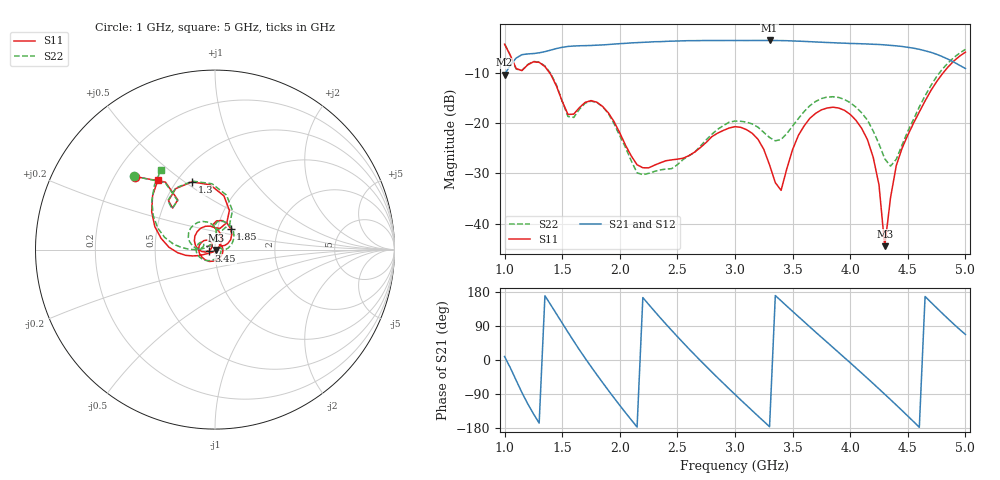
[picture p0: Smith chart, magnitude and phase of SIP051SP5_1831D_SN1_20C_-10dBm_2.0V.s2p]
# GHz  S  dB  R  50
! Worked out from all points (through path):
!   81 points, 1 GHz to 5 GHz, reference 50 ohm
!   highest |S21| = -3.65 dB at 3.3 GHz (marker M1); lowest = -10.4 dB at 1 GHz (marker M2)
!   lowest |S11| = -44.4 dB at 4.3 GHz (marker M3), VSWR 1.01, Z = 50.5 - j0.265 ohm
!   |S11| at or under -10 dB: 1.388 GHz to 4.81 GHz (3.421 GHz wide, 110 % of centre)
!   |S22| runs from -30.3 to -4.3 dB; largest |S21 - S12| = 0.0028
!   S11 on the Smith chart (normalised r, x): 1 GHz: 0.28, +0.36; 1.3 GHz: 0.59, +0.53; 1.85 GHz: 1.15, +0.28; 3.45 GHz: 0.93, -0.01; 5 GHz: 0.40, +0.41
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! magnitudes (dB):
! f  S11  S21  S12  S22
! 1 GHz  -4.4  -10.4  -10.4  -4.3
! 1.1 GHz  -9.2  -7.1  -7.1  -9.3
! 1.3 GHz  -8.0  -6.1  -6.1  -7.9
! 1.55 GHz  -18.3  -4.8  -4.8  -18.7
! 1.7 GHz  -15.9  -4.7  -4.7  -16.1
! 1.85 GHz  -16.7  -4.5  -4.5  -16.7
! 2.15 GHz  -28.3  -4.1  -4.1  -29.9
! 2.35 GHz  -27.9  -3.9  -3.9  -29.3
! 3 GHz  -20.7  -3.7  -3.6  -19.6
! 3.2 GHz  -23.2  -3.7  -3.7  -20.8
! 3.3 GHz  -28.3  -3.6  -3.7  -22.9
! 3.4 GHz  -33.4  -3.7  -3.7  -23.3
! 3.45 GHz  -29.1  -3.7  -3.7  -22.1
! 3.7 GHz  -18.1  -3.9  -3.9  -15.7
! 3.9 GHz  -17.0  -4.2  -4.2  -14.9
! 4.1 GHz  -21.1  -4.3  -4.3  -18.0
! 4.25 GHz  -32.3  -4.4  -4.5  -24.2
! 4.3 GHz  -44.4  -4.5  -4.5  -27.1
! 4.35 GHz  -34.8  -4.6  -4.6  -28.6
! 4.45 GHz  -25.0  -4.8  -4.8  -24.4
! 4.6 GHz  -17.8  -5.4  -5.4  -16.8
! 5 GHz  -6.0  -9.2  -9.2  -5.4
